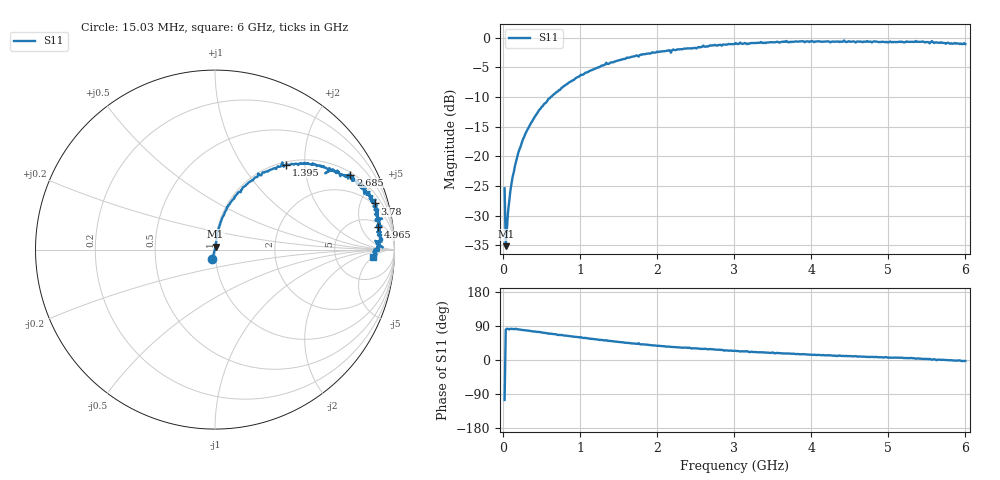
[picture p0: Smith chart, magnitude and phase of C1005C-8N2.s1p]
!	Network	Analyzer	HP8753E.07.74:	Oct	30	2002	Serial	No.	JP38451487
!	Hewlett-Packard
!	7	Sep	2009	8:35:42
!	Frequency	S11
#	HZ	S	RI	R	50
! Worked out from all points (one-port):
!   400 points, 15.03 MHz to 6 GHz, reference 50 ohm
!   lowest |S11| = -35.2 dB at 30.03 MHz (marker M1), VSWR 1.04, Z = 50.3 + j1.73 ohm
!   |S11| at or under -10 dB: start of sweep to 615.3 MHz
!   S11 on the Smith chart (normalised r, x): 15.03 MHz: 0.97, -0.10; 1.395 GHz: 1.05, +1.61; 2.685 GHz: 1.09, +3.55; 3.78 GHz: 1.83, +6.56; 4.965 GHz: 7, +10; 6 GHz: 14, -5
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1.502992e7  -0.0143 -0.0517
3.002985e7  0.00295 0.0172
6.00297e7  0.00465 0.0339
1.050295e8  0.00826 0.0587
1.500292e8  0.0122 0.0823
2.400288e8  0.0239 0.129
4.650277e8  0.0666 0.237
7.650262e8  0.156 0.347
1.005025e9  0.24 0.424
1.395023e9  0.397 0.474
1.515022e9  0.439 0.473
2.265019e9  0.664 0.442
2.685017e9  0.754 0.418
2.865016e9  0.795 0.364
3.015015e9  0.821 0.369
3.165014e9  0.808 0.35
3.195014e9  0.832 0.311
3.765011e9  0.881 0.264
3.780011e9  0.889 0.257
4.515007e9  0.909 0.164
4.965005e9  0.907 0.124
5.265004e9  0.92 0.0797
5.535002e9  0.893 0.0489
5.565002e9  0.935 0.0121
5.595002e9  0.9 0.0353
5.625002e9  0.913 -0.0076
5.655002e9  0.906 0.0167
6e9  0.882 -0.04
